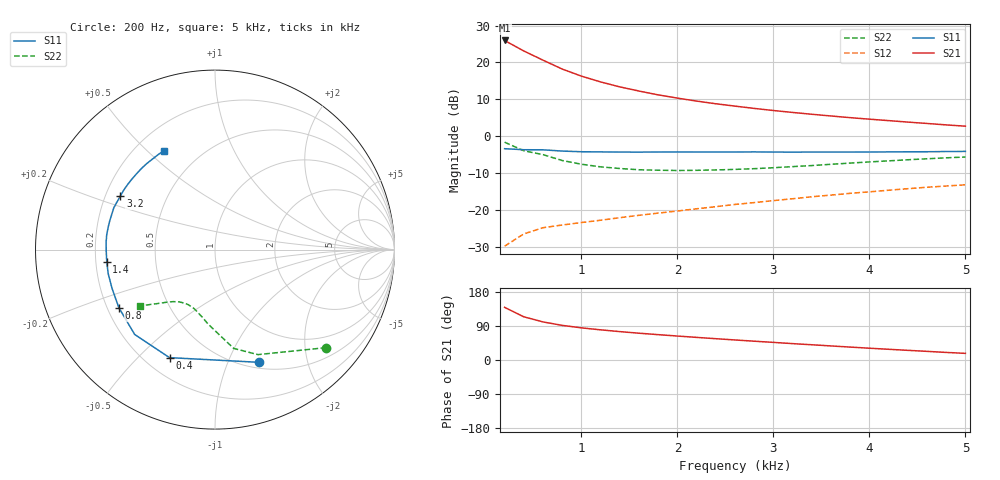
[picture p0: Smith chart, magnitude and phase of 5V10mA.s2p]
#  HZ  S  MA  R  50.0000
! Device:MCH4020
! Bias:VCE=5V, IC=10mA
!MHZ	S11(MAG/ANG)		S21(MAG/ANG)		S12(MAG/ANG)		S22(MAG/ANG)
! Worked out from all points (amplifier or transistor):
!   25 points, 200 Hz to 5 kHz, reference 50 ohm
!   highest |S21| = 26.0 dB at 200 Hz (marker M1)
!   |S21| within 3 dB of that: start of sweep to 411.4 Hz
!   unconditionally stable (mu >= 1): 2.686 kHz to 3.525 kHz
!   at 1 kHz: K = 0.58, MSG = 19.9 dB, |S12| = -23.5 dB
!   at 2.6 kHz: K = 1.00, MSG = 13.4 dB, |S12| = -18.6 dB
!   at 5 kHz: K = 0.91, MSG = 8.0 dB, |S12| = -13.2 dB
!   S11 on the Smith chart (normalised r, x): 200 Hz: 0.57, -1.30; 400 Hz: 0.30, -0.62; 800 Hz: 0.25, -0.26; 1.4 kHz: 0.25, -0.05; 3.2 kHz: 0.26, +0.25; 5 kHz: 0.32, +0.57
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200  0.674 -68.7  19.89 138.9  0.032 61.8  0.826 -41.4
400  0.653 -112.8  14.32 114.0  0.047 49.2  0.632 -67.8
600  0.651 -133.4  10.74 100.5  0.057 45.9  0.56 -79.3
800  0.626 -148.8  8.133 91.4  0.062 45.3  0.466 -88.2
1000  0.613 -159.3  6.522 84.8  0.067 46.0  0.415 -95.5
1200  0.61 -167.2  5.44 79.6  0.072 47.5  0.382 -100.9
1400  0.607 -173.5  4.659 74.9  0.078 48.7  0.363 -105.3
1600  0.606 -179.1  4.091 70.7  0.084 50.5  0.349 -109.4
1800  0.608 176.2  3.63 66.9  0.09 51.6  0.344 -112.7
2000  0.609 172.2  3.28 63.2  0.096 52.7  0.341 -116.0
2200  0.608 168.1  2.988 59.7  0.103 53.5  0.343 -118.8
2400  0.608 164.5  2.749 56.2  0.11 54.2  0.347 -121.6
2600  0.608 160.9  2.553 52.9  0.118 54.6  0.353 -124.4
2800  0.61 157.5  2.377 49.6  0.125 54.9  0.361 -126.4
3000  0.607 154.0  2.225 46.5  0.133 54.9  0.372 -128.8
3200  0.606 150.5  2.095 43.2  0.141 54.9  0.385 -130.8
3400  0.607 146.9  1.979 40.2  0.15 54.6  0.398 -132.6
3800  0.607 139.7  1.78 34.1  0.167 53.6  0.43 -136.0
4200  0.61 132.0  1.623 28.3  0.184 52.1  0.461 -138.8
4600  0.613 124.5  1.484 22.8  0.202 50.1  0.492 -141.1
4800  0.617 120.7  1.419 20.0  0.21 49.1  0.507 -142.0
5000  0.62 117.1  1.364 17.5  0.218 48.0  0.52 -143.0
